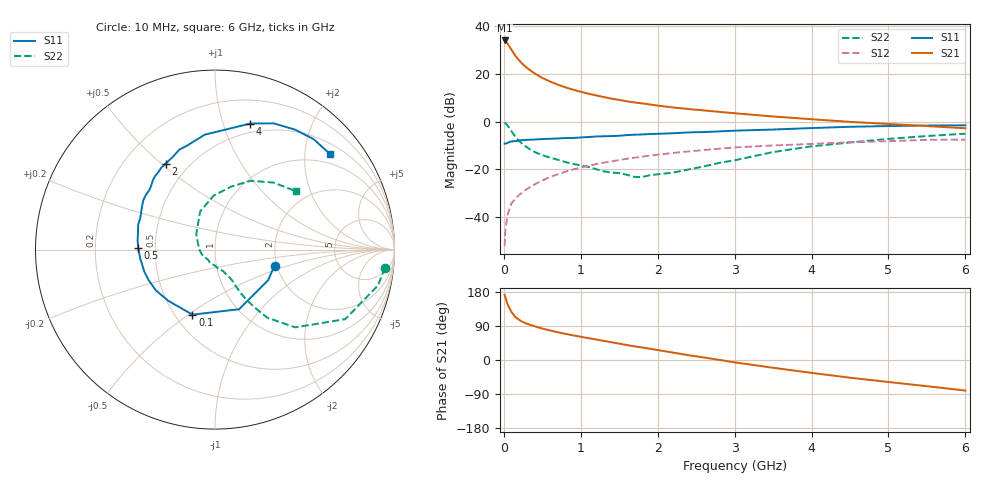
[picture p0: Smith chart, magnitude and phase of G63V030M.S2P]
! SIEMENS Small Signal Semiconductors
! BFG193
! Si NPN RF Bipolar Junction Transistor in SOT223
! VCE = 3 V  IC = 30 mA
! Common Emitter S-Parameters:  August  1996
# GHz  S  MA  R  50
!  f  S11  S21  S12  S22
! GHz  MAG  ANG  MAG  ANG  MAG  ANG  MAG  ANG
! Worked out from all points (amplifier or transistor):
!   36 points, 10 MHz to 6 GHz, reference 50 ohm
!   highest |S21| = 34.1 dB at 10 MHz (marker M1)
!   |S21| within 3 dB of that: start of sweep to 81.4 MHz
!   unconditionally stable (mu >= 1): 579.4 MHz to 2.407 GHz
!   at 250 MHz: K = 0.84, MSG = 26.8 dB, |S12| = -29.5 dB
!   at 1.4 GHz: K = 1.05, MAG = 11.8 dB, |S12| = -16.7 dB
!   at 6 GHz: K = 0.90, MSG = 2.4 dB, |S12| = -7.6 dB
!   S11 on the Smith chart (normalised r, x): 10 MHz: 1.94, -0.39; 100 MHz: 0.61, -0.52; 500 MHz: 0.40, +0.01; 2 GHz: 0.37, +0.52; 4 GHz: 0.41, +1.23; 6 GHz: 0.74, +2.58
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0.01  0.3437 -15.0  50.62 172.1  0.0024 86.3  0.9515 -6.1
0.02  0.3418 -29.9  49.28 165.5  0.0052 83.2  0.9298 -12.4
0.05  0.3583 -68.0  43.16 146.2  0.0114 71.7  0.8227 -28.1
0.1  0.3836 -109.1  32.1 126.5  0.0191 64.4  0.6225 -44.1
0.15  0.3867 -132.8  24.12 113.4  0.0241 62.0  0.4782 -52.5
0.2  0.4005 -145.7  19.27 105.9  0.0288 62.7  0.3907 -55.6
0.25  0.4072 -155.5  15.81 100.0  0.0334 63.1  0.3261 -58.0
0.3  0.4125 -162.4  13.41 95.7  0.0382 64.0  0.2868 -59.3
0.4  0.4191 -172.8  10.26 89.0  0.0478 65.2  0.2291 -60.4
0.5  0.4287 178.9  8.25 82.9  0.0576 64.4  0.1956 -60.9
0.6  0.4345 172.9  6.945 78.0  0.0682 64.1  0.1747 -62.4
0.8  0.4502 162.0  5.233 69.1  0.0878 61.6  0.1408 -67.1
1.1  0.4722 149.4  3.848 57.7  0.1174 56.9  0.1108 -79.3
1.6  0.5192 131.8  2.659 39.4  0.1648 46.6  0.076 -114.3
2  0.5526 119.8  2.164 26.2  0.2008 37.9  0.0778 -159.6
2.2  0.5673 114.5  1.976 19.5  0.2187 33.4  0.0844 -175.7
2.8  0.6206 99.5  1.595 0.3  0.2694 19.7  0.135 140.7
3.5  0.6791 83.1  1.278 -20.5  0.3144 2.5  0.2283 111.2
4  0.7292 74.4  1.118 -34.0  0.3379 -7.3  0.3009 91.4
4.5  0.7756 65.1  0.984 -46.7  0.3681 -17.4  0.363 75.5
5.5  0.8249 48.3  0.803 -69.1  0.4123 -40.6  0.4962 48.8
6  0.8332 39.8  0.723 -80.6  0.4176 -54.0  0.555 36.0
